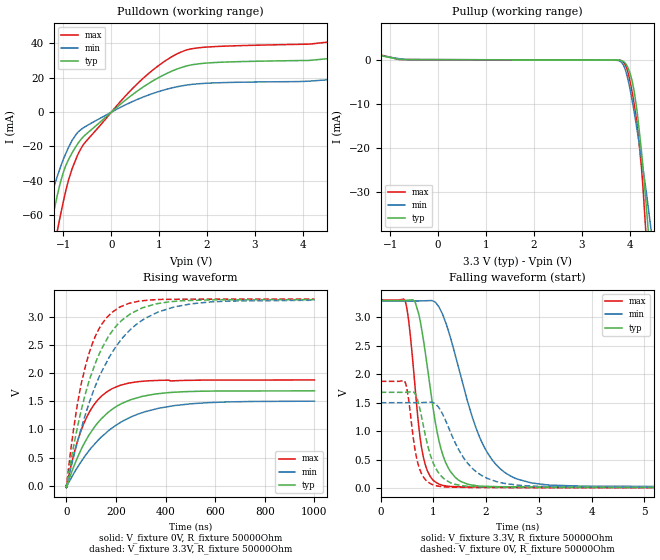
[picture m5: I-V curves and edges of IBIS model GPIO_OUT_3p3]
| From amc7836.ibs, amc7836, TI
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|   Model
[Model]   GPIO_OUT_3p3
Model_type   Output
Polarity   Non-Inverting
Vmeas = 1.65
Vref = 0
Cref = 1pF
Rref = 100000
|   typ   min   max
C_comp   2.855pF   2.622pF   2.914pF
[Voltage Range]   3.3   3.29   3.31
[Temperature Range]   27   125   -40
[Pullup Reference]   3.3   3.29   3.31
[Pulldown Reference]   0   0   0
[Power Clamp Reference]   3.3   3.29   3.31
[GND Clamp Reference]   0   0   0
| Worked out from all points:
|   slope of the pulldown table from 0 to 0.495 V, typ, clamps not added: 43.8 ohm
|   slope of the pullup table from 0 to 0.495 V, typ, clamps not added: 48 kohm
|   falling waveform, V_fixture 3.3V, R_fixture 50000Ohm: 20-80 % time 347ps typ, 672ps min, 218ps max; typ from 3.3 V to 0.005 V
|   rising waveform, V_fixture 0V, R_fixture 50000Ohm: 20-80 % time 152ns typ, 210ns min, 103ns max; typ from 0.003 V to 1.68 V
|   rising waveform, V_fixture 3.3V, R_fixture 50000Ohm: 20-80 % time 141ns typ, 190ns min, 97.8ns max; typ from 0.005 V to 3.3 V
|   falling waveform, V_fixture 0V, R_fixture 50000Ohm: 20-80 % time 296ps typ, 567ps min, 186ps max; typ from 1.68 V to 0.003 V
[Pulldown]
|   Voltage   I(typ)   I(min)   I(max)
-3.3V     -418.2mA   -289.2mA   -553.7mA
-1.478V   -99.98mA   -71.19mA   -136.8mA
-1.27V    -68.14mA   -50.55mA   -93.25mA
-1.132V   -48.99mA   -37.79mA   -69.82mA
-993.3mV  -34.47mA   -26.95mA   -51.09mA
-815.1mV  -23.58mA   -16.31mA   -32.73mA
-577.5mV  -14.21mA   -9.069mA   -18.78mA
551.1mV   12.39mA    7.448mA    16.7mA
1.403V    25.36mA    14.9mA     34.32mA
1.996V    28.55mA    16.79mA    37.85mA
4.145V    30.09mA    18.03mA    39.56mA
6.6V      37.57mA    23.52mA    49.12mA
[Pullup]
|   Voltage   I(typ)   I(min)   I(max)
-3.3V     5.688mA    4.803mA    6.793mA
-815.1mV  51.97uA    223.1uA    30.18uA
3.828V    -215.4uA   -607.1uA   -260.3uA
3.947V    -1.501mA   -3.823mA   -2.369mA
4.026V    -3.889mA   -7.875mA   -6.082mA
4.085V    -6.849mA   -11.53mA   -9.757mA
4.165V    -12.85mA   -16.8mA    -15.77mA
4.244V    -20.79mA   -22.33mA   -24.49mA
4.343V    -33.01mA   -29.92mA   -40.41mA
4.353V    -34.32mA   -30.73mA   -42.24mA
4.452V    -48.12mA   -39.25mA   -61.82mA
6.6V      -417.9mA   -290.3mA   -551mA
[Ramp]
R_load = 50000
|   typ   min   max
dV/dt_r   1.00861/1.5217e-07   0.898442/2.10397e-07   1.12453/1.02793e-07
dV/dt_f   1.97696/3.47154e-10   1.9695/6.71712e-10   1.98335/2.18173e-10
[Falling Waveform]
V_fixture = 3.3V
V_fixture_min = 3.29V
V_fixture_max = 3.31V
R_fixture = 50000Ohm
C_fixture = 0F
|   Time   V(typ)   V(min)   V(max)
0s        3.3V       3.29V      3.31V
472.8ps   3.3V       3.29V      3.263V
558.2ps   3.308V     3.29V      2.718V
724.1ps   3.054V     3.29V      1.068V
942.7ps   1.742V     3.298V     198.6mV
1.156ns   650.2mV    3.093V     52.9mV
1.414ns   187.2mV    2.34V      24mV
1.96ns    30.51mV    727.4mV    14.54mV
2.594ns   20.99mV    156.2mV    10.46mV
1us       5.271mV    7.821mV    4.415mV
[Rising Waveform]
V_fixture = 0V
V_fixture_min = 0V
V_fixture_max = 0V
R_fixture = 50000Ohm
C_fixture = 0F
|   Time   V(typ)   V(min)   V(max)
0s        2.654mV    3.536mV    2.465mV
558.2ps   -17.16mV   2.868mV    -35.88mV
20.01ns   220.8mV    138.2mV    373mV
41.94ns   466.7mV    304.6mV    741mV
80.87ns   817.7mV    560.1mV    1.203V
130.8ns   1.136V     819.2mV    1.541V
184.4ns   1.355V     1.024V     1.722V
307ns     1.587V     1.298V     1.853V
434.8ns   1.659V     1.422V     1.863V
1us       1.684V     1.501V     1.877V
[Rising Waveform]
V_fixture = 3.3V
V_fixture_min = 3.29V
V_fixture_max = 3.31V
R_fixture = 50000Ohm
C_fixture = 0F
|   Time   V(typ)   V(min)   V(max)
0s        5.271mV    7.821mV    4.415mV
41.94ns   970mV      724.9mV    1.362V
62.26ns   1.372V     1.045V     1.847V
80.87ns   1.692V     1.315V     2.18V
130.8ns   2.316V     1.912V     2.774V
184.4ns   2.739V     2.359V     3.076V
288.8ns   3.117V     2.884V     3.271V
434.8ns   3.27V      3.171V     3.307V
653.2ns   3.299V     3.276V     3.309V
1us       3.3V       3.29V      3.31V
[Falling Waveform]
|Gnd
V_fixture = 0V
V_fixture_min = 0V
V_fixture_max = 0V
R_fixture = 50000Ohm
C_fixture = 0F
|   Time   V(typ)   V(min)   V(max)
0s        1.684V     1.501V     1.877V
460.2ps   1.683V     1.501V     1.868V
506.8ps   1.687V     1.501V     1.694V
682.5ps   1.595V     1.501V     523.1mV
913.4ps   674.6mV    1.509V     93.88mV
1.192ns   170mV      1.265V     21.6mV
1.477ns   52.71mV    678.5mV    12.66mV
1.812ns   21.82mV    285.3mV    9.104mV
2.951ns   11.56mV    31.88mV    5.658mV
1us       2.654mV    3.536mV    2.465mV
